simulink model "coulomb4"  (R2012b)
settings: Solver=ode45  StartTime=0.0  StopTime=10.0  RelTol=1e-3
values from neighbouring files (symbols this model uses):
  c = 2200    [coulomb_1.m]    (also in coulomb_10.m = 0.1; coulomb_11.m = 0; coulomb_2.m; coulomb_3.m)
  Fex_ampl = 800    [coulomb_1.m]    (also in coulomb_2.m; coulomb_3.m; coulomb_4.m; coulomb_5.m)
  FG = 500    [coulomb_1.m]    (also in coulomb_10.m = 10; coulomb_11.m = 10; coulomb_2.m; coulomb_3.m)
  FH = 12    [coulomb_10.m]    (also in coulomb_11.m; coulomb_3.m = 600; coulomb_4.m = 600; position_reg_1.m = 3.956)
  fu = 0.02    [coulomb_1.m]    (also in coulomb_2.m; coulomb_3.m; coulomb_4.m; coulomb_5.m = 0.1)
  m = 400    [coulomb_1.m]    (also in coulomb_10.m = 10; coulomb_11.m = 10; coulomb_2.m; coulomb_3.m)
  v0 = 0    [coulomb_1.m]    (also in coulomb_2.m; coulomb_3.m; coulomb_4.m; coulomb_5.m)
  vstr = 0.1    [coulomb_10.m]    (also in coulomb_11.m; coulomb_3.m = 0.05; coulomb_4.m = 0.01; slip_stick_1.m = 0.01)
  y0 = 0    [coulomb_1.m]    (also in coulomb_2.m; coulomb_3.m; coulomb_4.m; coulomb_5.m)
undefined symbols (not defined in the file or in its folder): sgn

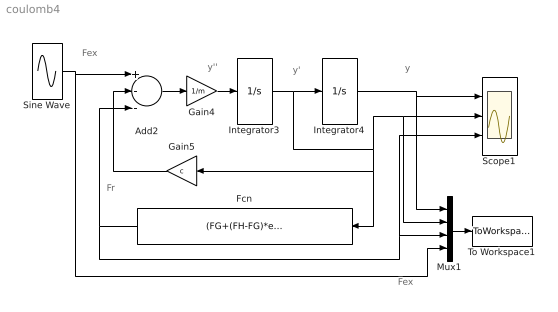
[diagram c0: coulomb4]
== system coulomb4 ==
  note: Fex
  note: Fr
  note: Fex
  note: y
  note: y'
  note: y''
  Add2 : Sum  Inputs=+--
  Fcn : Fcn  Expr=(FG+(FH-FG)*exp(-abs(u)/vstr))*sgn(u)
  Gain4 : Gain  Gain=1/m
  Gain5 : Gain  Gain=c
  Integrator3 : Integrator  InitialCondition=v0
  Integrator4 : Integrator  InitialCondition=y0
  Mux1 : Mux
  Scope1 : Scope  NumInputPorts=3
  Sine Wave : Sin  Amplitude=Fex_ampl  Frequency=2*pi*fu  SampleTime=0
  To Workspace1 : ToWorkspace  VariableName=y  SampleTime=-1  SaveFormat=Structure With Time
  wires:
  Add2/1 -> Gain4/1
  Gain4/1 -> Integrator3/1
  Gain5/1 -> Add2/2
  Integrator4/1 -> Scope1/1, Mux1/1
  Integrator3/1 -> Fcn/1, Gain5/1, Scope1/2, Mux1/2, Integrator4/1
  Fcn/1 -> Add2/3, Mux1/3, Scope1/3
  Mux1/1 -> To Workspace1/1
  Sine Wave/1 -> Mux1/4, Add2/1
